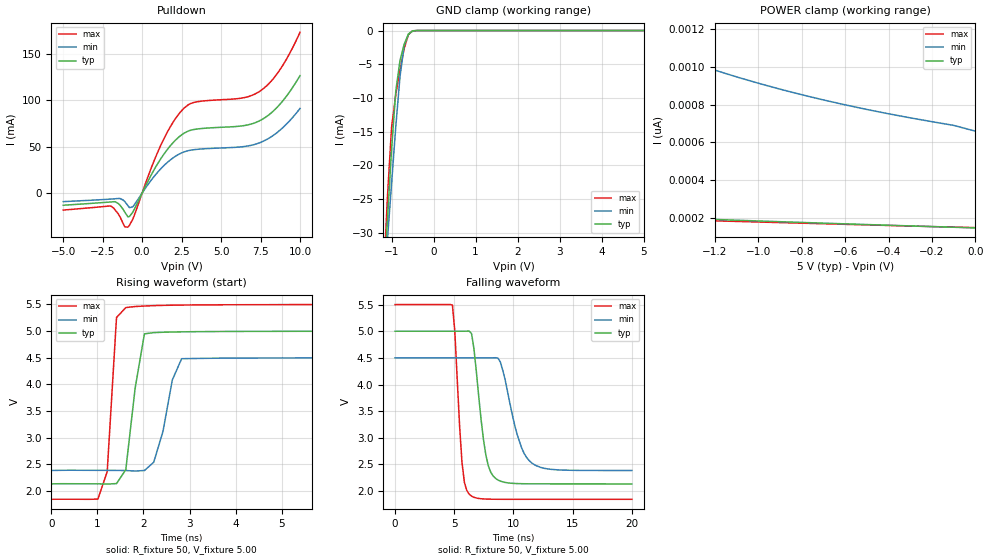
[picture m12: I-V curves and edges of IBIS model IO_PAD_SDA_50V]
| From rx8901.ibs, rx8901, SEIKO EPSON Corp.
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[Model]   IO_PAD_SDA_50V
Model_type I/O_open_drain
Enable Active-High
Polarity Non-Inverting
Vinh=3.50
Vinl=1.50
Vref=5.50
Vmeas=2.50
Rref=5000
C_comp   2.5p   2.0p   3.0p
[Temperature Range] 25   105   -40
[Voltage Range]   5.00   4.50   5.50
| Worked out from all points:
|   slope of the pulldown table from 0 to 0.75 V, typ, clamps not added: 30.2 ohm
|   GND clamp passes 1 mA (typ) near -0.63 V on its own axis
|   falling waveform, R_fixture 50, V_fixture 5.00: 20-80 % time 869ps typ, 1.39ns min, 543ps max; typ from 5 V to 2.14 V
|   rising waveform, R_fixture 50, V_fixture 5.00: 20-80 % time 260ps typ, 309ps min, 153ps max; typ from 2.14 V to 5 V
[Pulldown]
-5V       -13.17mA   -9.276mA   -18.36mA
-2V       -9.661mA   -6.552mA   -13.89mA
-1.5V     -11.48mA   -5.908mA   -22.8mA
-1.1V     -20.65mA   -9.218mA   -36.45mA
-900mV    -25.65mA   -13.69mA   -36.75mA
-600mV    -20.79mA   -14.97mA   -28.48mA
1.1V      34.77mA    24.59mA    48.37mA
2.4V      61.28mA    42.36mA    86.7mA
3.3V      68.39mA    46.65mA    97.55mA
7.4V      77.39mA    53.78mA    108.9mA
8.6V      93.1mA     65.74mA    129.5mA
10V       126.3mA    90.97mA    172.9mA
[GND Clamp]
-5V       -506.4mA   -413.5mA   -621mA
-1.2V     -38.91mA   -39.62mA   -38.2mA
-1.1V     -28.19mA   -31.12mA   -24.82mA
-1V       -17.59mA   -22.65mA   -14.32mA
-900mV    -8.974mA   -14.24mA   -9.514mA
-800mV    -4.446mA   -6.842mA   -5.831mA
-700mV    -2.032mA   -2.215mA   -2.664mA
-600mV    -545.2uA   -526uA     -623.9uA
-500mV    -56.87uA   -82.5uA    -37.95uA
5V        146.4pA    774pA      131.9pA
[POWER Clamp]
-5V       431.4pA    5.498nA    307.4pA
-4.3V     368.3pA    4.006nA    281.2pA
-3.5V     309.6pA    2.75nA     255.5pA
-2.7V     261.6pA    1.879nA    230.5pA
-1.7V     212.5pA    1.199nA    199.4pA
-1.6V     208.1pA    1.15nA     196.3pA
-1.3V     195.4pA    1.02nA     187pA
-1.1V     187.2pA    946.5pA    180.9pA
-900mV    179.4pA    881.5pA    174.7pA
-600mV    168pA      798.4pA    165.5pA
-100mV    150pA      689.6pA    150.7pA
0V        146.4pA    659pA      148pA
[Falling Waveform]
R_fixture=50
V_fixture=5.00
V_fixture_min=4.50
V_fixture_max=5.50
0s        5V         4.5V       5.5V
4.848ns   5V         4.5V       5.49V
5.051ns   5V         4.5V       4.996V
5.657ns   5V         4.5V       2.536V
6.465ns   4.954V     4.5V       1.906V
7.677ns   2.67V      4.5V       1.851V
8.485ns   2.24V      4.503V     1.848V
10.51ns   2.14V      2.934V     1.847V
11.52ns   2.137V     2.534V     1.847V
20ns      2.136V     2.387V     1.846V
[Rising Waveform]
R_fixture=50
V_fixture=5.00
V_fixture_min=4.50
V_fixture_max=5.50
0s        2.136V     2.387V     1.846V
1.01ns    2.136V     2.389V     1.85V
1.212ns   2.131V     2.389V     2.365V
1.414ns   2.141V     2.388V     5.256V
1.616ns   2.402V     2.385V     5.442V
1.818ns   3.928V     2.376V     5.462V
2.02ns    4.95V      2.386V     5.471V
2.222ns   4.972V     2.541V     5.479V
2.828ns   4.987V     4.483V     5.489V
20ns      5V         4.5V       5.5V
[Ramp]
R_load=50
dV/dt_r   1.719E+0/1.934E-10   1.268E+0/2.858E-10   2.192E+0/1.449E-10
dV/dt_f   1.719E+0/8.644E-10   1.268E+0/1.385E-9   2.192E+0/5.369E-10
|[End   IO_PAD_SDA_50V
